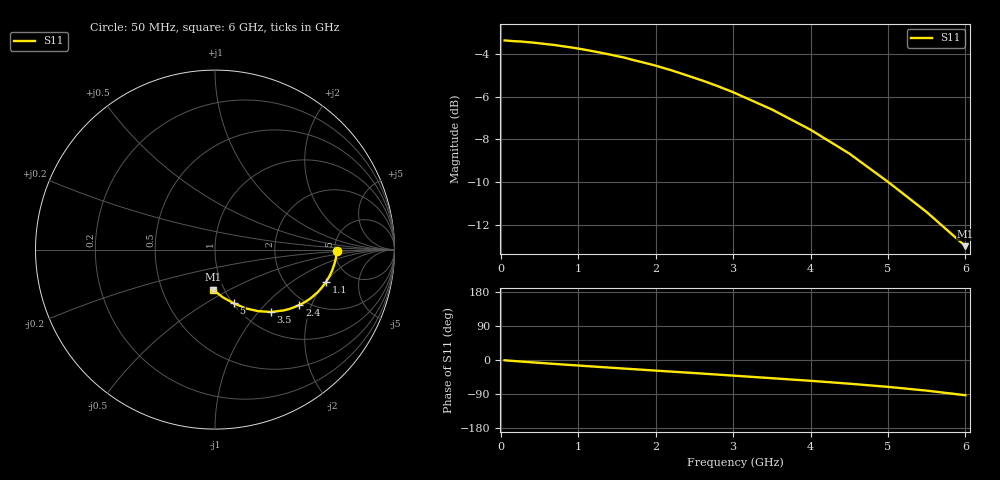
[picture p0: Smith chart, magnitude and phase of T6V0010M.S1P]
! SIEMENS Discrete & RF Semiconductors
! BAT62
! Si Schottky Diode in SOT143
! IF = 10 mA
! S-Parameters:  February  1997
# GHz  S  MA  R  50
!  f  S11
! GHz  MAG  ANG
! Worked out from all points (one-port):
!   34 points, 50 MHz to 6 GHz, reference 50 ohm
!   lowest |S11| = -13.0 dB at 6 GHz (marker M1), VSWR 1.58, Z = 44.3 - j20.8 ohm
!   |S11| at or under -10 dB: 5.002 GHz to end of sweep
!   S11 on the Smith chart (normalised r, x): 50 MHz: 5.22, -0.16; 1.1 GHz: 3.32, -2.02; 2.4 GHz: 1.82, -1.64; 3.5 GHz: 1.32, -1.17; 5 GHz: 1.01, -0.67; 6 GHz: 0.89, -0.42
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0.05  0.6789 -0.7
0.1  0.678 -1.6
0.15  0.6767 -2.4
0.25  0.6753 -3.9
0.4  0.6714 -6.1
0.5  0.6685 -7.5
0.6  0.6651 -9.0
0.7  0.6622 -10.4
0.8  0.658 -11.8
0.9  0.6542 -13.2
1  0.6498 -14.5
1.1  0.6451 -16.0
1.3  0.6349 -18.7
1.5  0.6239 -21.4
1.6  0.6186 -22.7
1.9  0.5991 -26.7
2  0.5926 -28.0
2.2  0.5781 -30.6
2.4  0.5625 -33.2
2.6  0.5471 -35.8
2.8  0.5307 -38.5
3  0.5134 -41.2
3.5  0.4678 -48.0
4  0.4193 -54.9
4.5  0.3688 -62.5
5  0.3164 -70.9
5.5  0.2688 -80.8
6  0.2236 -93.0
